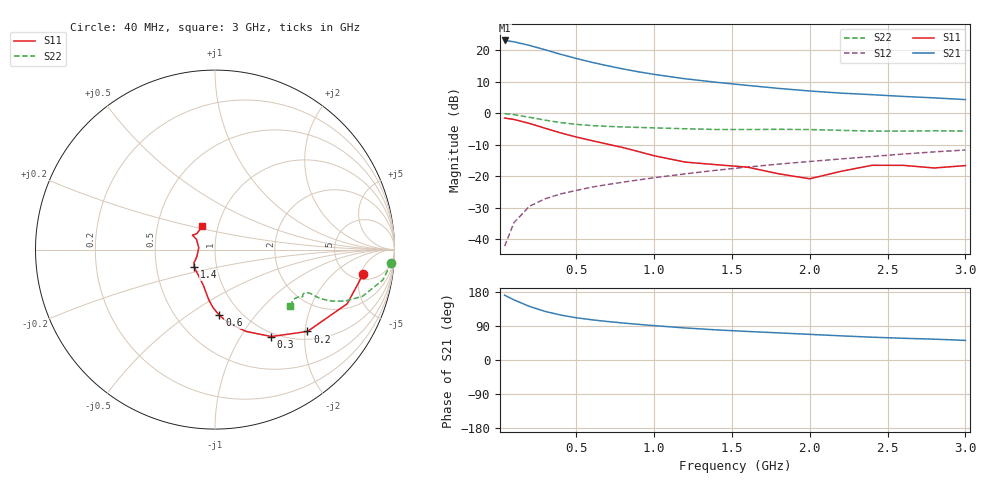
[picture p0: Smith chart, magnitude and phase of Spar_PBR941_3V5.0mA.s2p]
! Filename:  PBR941D.S2P  Version:  3.0
! NXP part #:  PBR941  Date: July 1998
! Bias condition:  Vce=3V, Ic=5.0mA
#  MHz  S  MA  R 50
! Freq  S11  S21  S12  S22
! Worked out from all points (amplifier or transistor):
!   21 points, 40 MHz to 3 GHz, reference 50 ohm
!   highest |S21| = 23.1 dB at 40 MHz (marker M1)
!   |S21| within 3 dB of that: start of sweep to 302.9 MHz
!   unconditionally stable (mu >= 1): 1.222 GHz to 2.531 GHz
!   at 300 MHz: K = 0.49, MSG = 23.7 dB, |S12| = -27.2 dB
!   at 1 GHz: K = 0.95, MSG = 16.4 dB, |S12| = -20.5 dB
!   at 3 GHz: K = 0.99, MSG = 8.0 dB, |S12| = -11.7 dB
!   S11 on the Smith chart (normalised r, x): 40 MHz: 6.23, -5.60; 200 MHz: 1.19, -2.06; 300 MHz: 0.95, -1.37; 600 MHz: 0.80, -0.67; 1.4 GHz: 0.78, -0.16; 3 GHz: 0.84, +0.22
40  0.838 -9.2  14.33 171.0  0.007714 85.2  0.9847 -4.3
100  0.7959 -22.3  13.63 158.7  0.01825 78.5  0.9502 -10.3
200  0.688 -41.5  11.96 141.4  0.03333 70.6  0.8616 -17.6
300  0.577 -57.1  10.19 128.2  0.04365 66.5  0.7755 -21.8
400  0.4867 -69.3  8.633 118.6  0.05223 65.2  0.7101 -23.8
500  0.4186 -79.1  7.416 111.5  0.0593 65.2  0.6654 -24.6
600  0.3669 -86.2  6.447 106.1  0.06693 65.8  0.6361 -24.9
700  0.3231 -92.0  5.682 101.6  0.07353 66.7  0.6178 -24.9
800  0.2845 -96.7  5.058 97.7  0.08026 67.9  0.6051 -24.8
900  0.2458 -101.6  4.549 94.0  0.08702 68.8  0.5949 -24.7
1000  0.211 -107.7  4.142 90.7  0.09439 69.8  0.5852 -24.7
1200  0.1673 -124.7  3.527 84.6  0.1087 71.0  0.5661 -25.1
1400  0.152 -140.0  3.102 79.5  0.1241 72.0  0.5517 -26.2
1600  0.1389 -147.6  2.767 75.3  0.1394 73.0  0.5503 -27.4
1800  0.1091 -158.4  2.48 71.6  0.1553 74.0  0.5547 -28.1
2000  0.09082 173.5  2.255 67.6  0.1711 74.2  0.5502 -28.6
2200  0.1192 150.6  2.086 63.8  0.1875 73.9  0.5343 -29.6
2400  0.1488 147.4  1.971 60.2  0.2051 73.9  0.5204 -31.7
2600  0.1484 147.6  1.849 57.3  0.2245 74.1  0.5195 -34.3
2800  0.1348 138.6  1.753 55.0  0.243 74.0  0.5256 -36.1
3000  0.1471 119.0  1.646 51.7  0.2601 73.3  0.5202 -36.8
